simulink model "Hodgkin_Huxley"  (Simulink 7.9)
settings: Solver=ode1  StartTime=0.0  StopTime=45  FixedStep=0.01  RelTol=1e-3
PreLoadFcn:
  | %This script has been adapted from Murat Saglam (22.4.2008) and his HH
  | %action potential simulink model to better represent the model shown in HP.
  | clear
  | 
  | gbarNa=120; gbarK=36; gbarL=.3; % conductance of ions in hypothetical situations
  | % where all gates in the channel are open:((muA/mV)/cm^2)
  | 
  | ENa=45; EK=-82; EL=-59; %Equilibrium potentials of ions: mV
  | 
  | n0=.3177; m0=.0529; h0=.5961; %initial number of gates open: (unitless)
  | 
  | t1p=20; t2p=21; % Beginning and ending current pulse: ms
  | ip=10;          % Amplitude of current pulse: muA
  | 
  | %Vhold = -70;   % resting membrane volate potential: mV
  | Vstart=-55;     % membrane voltage potential after initial current applied: mV
  | C = 1;          % membrane capacitance per unit area: (muF/cm^2)

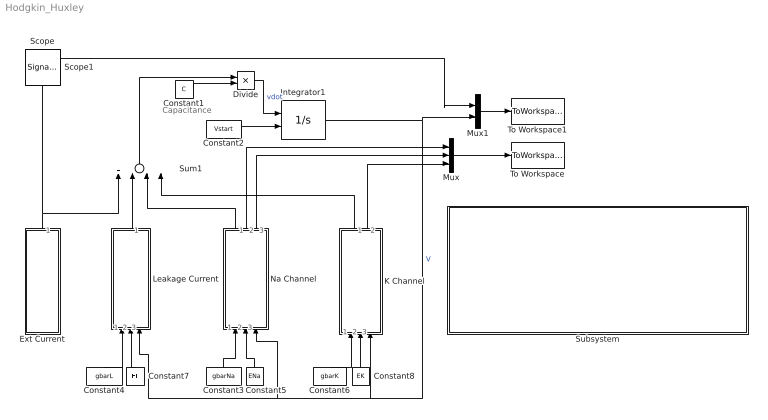
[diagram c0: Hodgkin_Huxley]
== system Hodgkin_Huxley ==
  note: Capacitance
  Constant1 : Constant  Value=C
  Constant2 : Constant  Value=Vstart
  Constant3 : Constant  Value=gbarNa
  Constant4 : Constant  Value=gbarL
  Constant5 : Constant  Value=ENa
  Constant6 : Constant  Value=gbarK
  Constant7 : Constant  Value=EL
  Constant8 : Constant  Value=EK
  Divide : Product  Inputs=*/
  Ext Current : Subsystem
  Integrator1 : Integrator  InitialConditionSource=external
  K Channel : Subsystem
  Leakage Current : Subsystem
  Mux : Mux  Inputs=3
  Mux1 : Mux  Inputs=2
  Na Channel : Subsystem
  Subsystem : Subsystem
  Sum1 : Sum  Inputs=+---
  To Workspace : ToWorkspace  VariableName=mhn  SampleTime=-1
  To Workspace1 : ToWorkspace  VariableName=I_V  SampleTime=-1  SaveFormat=Structure With Time
  Scope : SignalViewerScope  IOType=viewer  RefreshTime=0.035000
  Scope1 : SignalViewerScope  IOType=viewer  RefreshTime=0.035000
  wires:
  Leakage Current/1(IL) -> Sum1/2
  Na Channel/1(INa) -> Sum1/3
  K Channel/1(IK) -> Sum1/4
  Constant2/1 -> Integrator1/2
  Constant6/1 -> K Channel/1(gbarK)
  Constant4/1 -> Leakage Current/1(gbarL)
  Constant7/1 -> Leakage Current/2(EL)
  Constant8/1 -> K Channel/2(EK)
  Integrator1/1 -> Leakage Current/3(V), Na Channel/3(V), K Channel/3(V), Mux1/2  "V"
  Sum1/1 -> Divide/1
  Divide/1 -> Integrator1/1  "vdot"
  Constant1/1 -> Divide/2
  Constant3/1 -> Na Channel/1(gbarNa)
  Constant5/1 -> Na Channel/2(ENa)
  Mux/1 -> To Workspace/1
  Na Channel/2(m) -> Mux/1
  Na Channel/3(h) -> Mux/2
  K Channel/2(n) -> Mux/3
  Ext Current/1(I external) -> Sum1/1, Mux1/1
  Mux1/1 -> To Workspace1/1

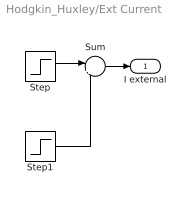
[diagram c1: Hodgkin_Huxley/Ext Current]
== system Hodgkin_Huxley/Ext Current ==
  Step : Step  Time=t1p  After=ip  SampleTime=0
  Step1 : Step  Time=t2p  After=-ip  SampleTime=0
  Sum : Sum  Inputs=|++
  I external : Outport
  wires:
  Step1/1 -> Sum/2
  Step/1 -> Sum/1
  Sum/1 -> I external/1

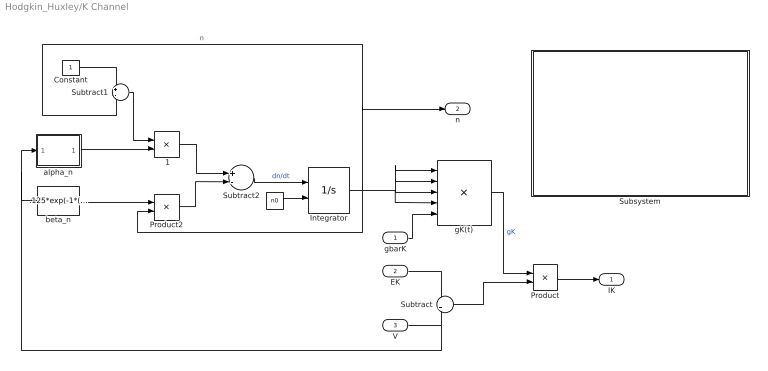
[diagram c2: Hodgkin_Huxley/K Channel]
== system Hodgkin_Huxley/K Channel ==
  gbarK : Inport
  EK : Inport  Port=2
  V : Inport  Port=3
  " " : Constant  Value=n0
  " 1" : Product
  Constant : Constant
  Integrator : Integrator  InitialConditionSource=external
  Product : Product
  Product2 : Product
  Subsystem : Subsystem
  Subtract : Sum  Inputs=-+
  Subtract1 : Sum  Inputs=+-
  Subtract2 : Sum  Inputs=+-
  alpha_n : Subsystem
  beta_n : Fcn  Expr=.125*exp(-1*((u+70)/80))
  gK(t) : Product  Inputs=5
  IK : Outport
  n : Outport  Port=2
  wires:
  EK/1 -> Subtract/1
  Constant/1 -> Subtract1/1
  alpha_n/1(Out1) -> " 1"/2
  beta_n/1 -> Product2/1
  Subtract1/1 -> " 1"/1
  Product2/1 -> Subtract2/2
  " 1"/1 -> Subtract2/1
  Subtract2/1 -> Integrator/1  "dn/dt"
  Integrator/1 -> Product2/2, gK(t)/3, gK(t)/4, gK(t)/2, gK(t)/1, Subtract1/2, n/1  "n"
  gbarK/1 -> gK(t)/5
  V/1 -> Subtract/2, beta_n/1, alpha_n/1(V)
  " "/1 -> Integrator/2
  gK(t)/1 -> Product/1  "gK"
  Subtract/1 -> Product/2
  Product/1 -> IK/1

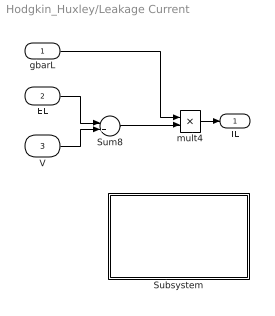
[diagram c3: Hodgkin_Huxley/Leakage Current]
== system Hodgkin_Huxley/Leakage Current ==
  gbarL : Inport
  EL : Inport  Port=2
  V : Inport  Port=3
  Subsystem : Subsystem
  Sum8 : Sum  Inputs=-+
  mult4 : Product  Inputs=**
  IL : Outport
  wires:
  Sum8/1 -> mult4/2
  gbarL/1 -> mult4/1
  EL/1 -> Sum8/1
  V/1 -> Sum8/2
  mult4/1 -> IL/1

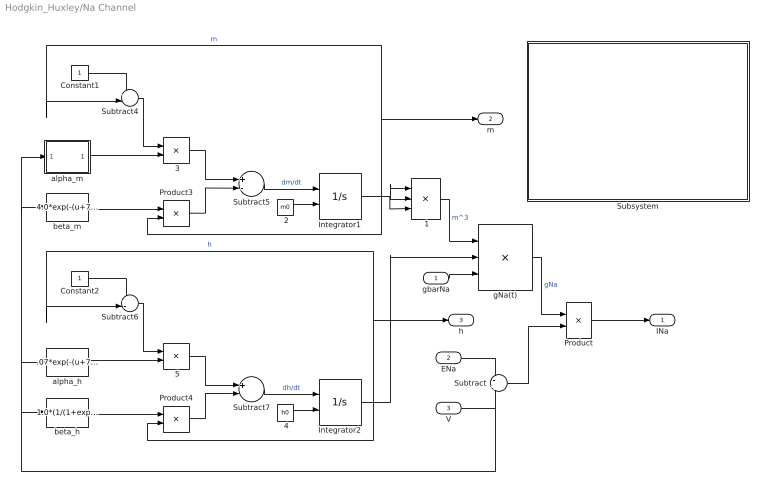
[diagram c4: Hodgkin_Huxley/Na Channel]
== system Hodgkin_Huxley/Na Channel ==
  gbarNa : Inport
  ENa : Inport  Port=2
  V : Inport  Port=3
  " 1" : Product  Inputs=3
  " 2" : Constant  Value=m0
  " 3" : Product
  " 4" : Constant  Value=h0
  " 5" : Product
  Constant1 : Constant
  Constant2 : Constant
  Integrator1 : Integrator  InitialConditionSource=external
  Integrator2 : Integrator  InitialConditionSource=external
  Product : Product
  Product3 : Product
  Product4 : Product
  Subsystem : Subsystem
  Subtract : Sum  Inputs=-+
  Subtract{4..7} (4 alike) : Sum  Inputs=+-
  alpha_h : Fcn  Expr=.07*exp(-(u+70)/20)
  alpha_m : Subsystem
  beta_h : Fcn  Expr=1.0*(1/(1+exp(-(u+40)/10)))
  beta_m : Fcn  Expr=4.0*exp(-(u+70)/18)
  gNa(t) : Product  Inputs=3
  INa : Outport
  m : Outport  Port=2
  h : Outport  Port=3
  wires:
  Constant1/1 -> Subtract4/1
  alpha_m/1(Out1) -> " 3"/2
  beta_m/1 -> Product3/1
  Subtract4/1 -> " 3"/1
  Product3/1 -> Subtract5/2
  " 3"/1 -> Subtract5/1
  Subtract5/1 -> Integrator1/1  "dm/dt"
  " 2"/1 -> Integrator1/2
  Constant2/1 -> Subtract6/1
  alpha_h/1 -> " 5"/2
  beta_h/1 -> Product4/1
  Subtract6/1 -> " 5"/1
  Product4/1 -> Subtract7/2
  " 5"/1 -> Subtract7/1
  Subtract7/1 -> Integrator2/1  "dh/dt"
  Integrator2/1 -> Product4/2, gNa(t)/2, Subtract6/2, h/1  "h"
  " 4"/1 -> Integrator2/2
  ENa/1 -> Subtract/1
  V/1 -> Subtract/2, beta_h/1, alpha_h/1, beta_m/1, alpha_m/1(Vstart)
  " 1"/1 -> gNa(t)/1  "m^3"
  gbarNa/1 -> gNa(t)/3
  Integrator1/1 -> Product3/2, " 1"/2, " 1"/1, " 1"/3, Subtract4/2, m/1  "m"
  gNa(t)/1 -> Product/1  "gNa"
  Subtract/1 -> Product/2
  Product/1 -> INa/1

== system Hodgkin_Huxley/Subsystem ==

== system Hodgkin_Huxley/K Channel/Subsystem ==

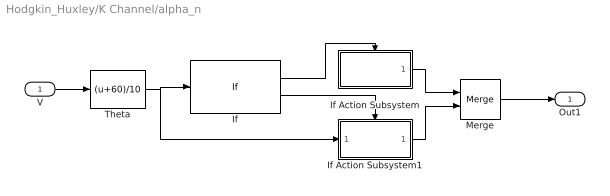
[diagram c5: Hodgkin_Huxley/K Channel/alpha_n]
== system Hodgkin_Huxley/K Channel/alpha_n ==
  V : Inport
  If : If  IfExpression=u1==0
  If Action Subsystem : Subsystem  TreatAsAtomicUnit=on
  If Action Subsystem1 : Subsystem  TreatAsAtomicUnit=on
  Merge : Merge
  Theta : Fcn  Expr=(u+60)/10
  Out1 : Outport
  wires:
  Theta/1 -> If/1, If Action Subsystem1/1(u1)
  V/1 -> Theta/1
  If Action Subsystem/1(Out1) -> Merge/1
  If Action Subsystem1/1(Out1) -> Merge/2
  If/1 -> If Action Subsystem/Action
  If/2 -> If Action Subsystem1/Action
  Merge/1 -> Out1/1

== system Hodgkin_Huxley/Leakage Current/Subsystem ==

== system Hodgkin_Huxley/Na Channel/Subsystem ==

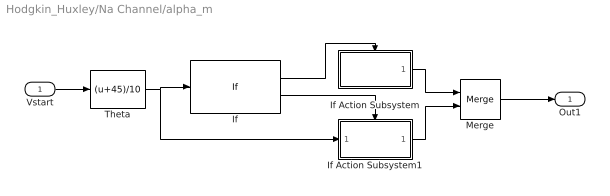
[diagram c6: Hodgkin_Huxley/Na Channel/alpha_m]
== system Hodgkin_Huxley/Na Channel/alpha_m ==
  Vstart : Inport
  If : If  IfExpression=u1==0
  If Action Subsystem : Subsystem  TreatAsAtomicUnit=on
  If Action Subsystem1 : Subsystem  TreatAsAtomicUnit=on
  Merge : Merge
  Theta : Fcn  Expr=(u+45)/10
  Out1 : Outport
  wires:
  Theta/1 -> If/1, If Action Subsystem1/1(u1)
  Vstart/1 -> Theta/1
  If Action Subsystem/1(Out1) -> Merge/1
  If Action Subsystem1/1(Out1) -> Merge/2
  If/1 -> If Action Subsystem/Action
  If/2 -> If Action Subsystem1/Action
  Merge/1 -> Out1/1

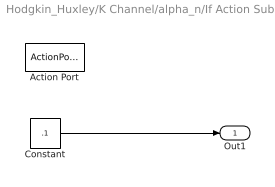
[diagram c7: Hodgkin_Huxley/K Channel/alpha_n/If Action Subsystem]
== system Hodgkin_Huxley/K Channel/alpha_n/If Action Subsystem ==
  Action Port : ActionPort  PropagateVarSize=During execution  ActionType=then
  Constant : Constant  Value=.1
  Out1 : Outport  InitialOutput=[.1]
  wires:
  Constant/1 -> Out1/1

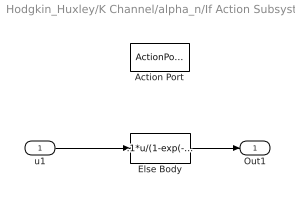
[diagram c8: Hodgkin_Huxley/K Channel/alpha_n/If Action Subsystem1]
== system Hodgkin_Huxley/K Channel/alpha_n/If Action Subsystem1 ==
  u1 : Inport
  Action Port : ActionPort  PropagateVarSize=During execution  ActionType=else
  Else Body : Fcn  Expr=.1*u/(1-exp(-u))
  Out1 : Outport
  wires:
  u1/1 -> Else Body/1
  Else Body/1 -> Out1/1

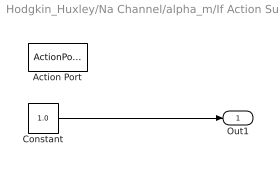
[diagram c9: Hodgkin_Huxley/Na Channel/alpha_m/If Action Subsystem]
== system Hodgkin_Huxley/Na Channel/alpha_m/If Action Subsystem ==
  Action Port : ActionPort  PropagateVarSize=During execution  ActionType=then
  Constant : Constant  Value=1.0
  Out1 : Outport  InitialOutput=[1.0]
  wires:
  Constant/1 -> Out1/1

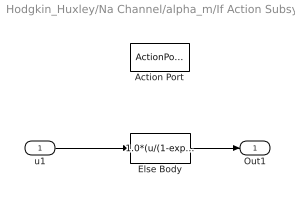
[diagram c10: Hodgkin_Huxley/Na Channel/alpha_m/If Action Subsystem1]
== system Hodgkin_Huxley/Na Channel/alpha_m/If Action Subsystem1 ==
  u1 : Inport
  Action Port : ActionPort  PropagateVarSize=During execution  ActionType=else
  Else Body : Fcn  Expr=1.0*(u/(1-exp(-u)))
  Out1 : Outport
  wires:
  u1/1 -> Else Body/1
  Else Body/1 -> Out1/1
